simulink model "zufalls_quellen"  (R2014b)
settings: Solver=ode45  StartTime=0.0  StopTime=10.0  RelTol=1e-3
libraries: simulink x1, dspsrcs4 x1

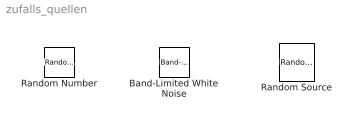
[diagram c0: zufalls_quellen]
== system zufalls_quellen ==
  Band-Limited White Noise : simulink/Sources/Band-Limited White Noise  Cov=[0.1]  Ts=0.1  seed=[23341]
  Random Number : RandomNumber  SampleTime=0.1
  Random Source : dspsrcs4/Random Source  SrcType=Uniform  NormMethod=Ziggurat  CltLength=12  MinVal=0  MaxVal=1  MeanVal=0  VarVal=1  RepMode=Specify seed  rawSeed=3679  IsInherit=off  SampMode=Discrete  SampTime=1/1000  SampFrame=1  DataType=Double  OutComplex=Real
